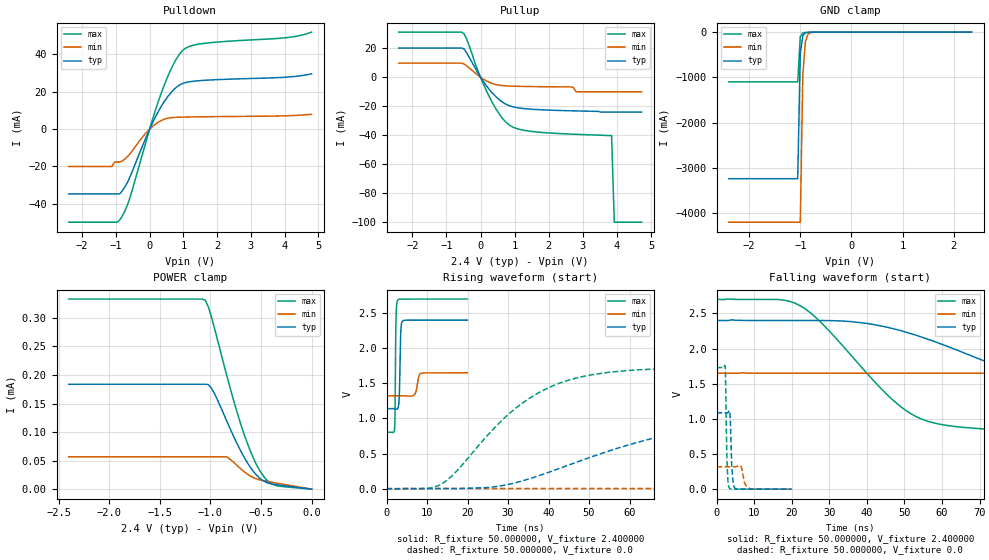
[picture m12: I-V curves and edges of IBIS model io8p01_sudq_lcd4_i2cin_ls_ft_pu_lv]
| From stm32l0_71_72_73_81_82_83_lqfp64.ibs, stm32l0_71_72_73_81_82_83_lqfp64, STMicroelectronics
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|   Model io8p01_sudq_lcd4_i2cin_ls_ft_pu_lv
[Model]  io8p01_sudq_lcd4_i2cin_ls_ft_pu_lv
Model_type I/O
Polarity   Non-Inverting
Enable   Active-Low
Vinl =   0.720000V
Vinh =   1.680000V
Vmeas =  1.200000V
Cref =   50.000000pF
Rref =   100.000000M
Vref =   0.0V
C_comp   2.470900pF   2.435200pF   2.490500pF
[Temperature Range]   25.000000   0.105000k   -40.000000
[Pullup Reference]   2.400000V   1.650000V   2.700000V
[Pulldown Reference]   0.0V   0.0V   0.0V
[POWER Clamp Reference]   2.400000V   1.650000V   2.700000V
[GND Clamp Reference]   0.0V   0.0V   0.0V
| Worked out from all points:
|   slope of the pulldown table from 0 to 0.36 V, typ, clamps not added: 28.5 ohm
|   slope of the pullup table from 0 to 0.36 V, typ, clamps not added: 32.2 ohm
|   GND clamp passes 1 mA (typ) near -0.64 V on its own axis
|   rising waveform, R_fixture 50.000000, V_fixture 2.400000: 20-80 % time 282ps typ, 636ps min, 192ps max; typ from 1.14 V to 2.4 V
|   rising waveform, R_fixture 50.000000, V_fixture 0.0: 20-80 % time 39.5ns typ, 107ns min, 19.3ns max; typ from 0.001 V to 1.09 V
|   falling waveform, R_fixture 50.000000, V_fixture 2.400000: 20-80 % time 40.8ns typ, 106ns min, 20.1ns max; typ from 2.4 V to 1.14 V
|   falling waveform, R_fixture 50.000000, V_fixture 0.0: 20-80 % time 457ps typ, 824ps min, 362ps max; typ from 1.09 V to 0.001 V
[Pulldown]
|Voltage   I(typ)   I(min)   I(max)
-2.4V     -34.71mA   -20mA      -49.82mA
-1.12V    -34.71mA   -20mA      -49.82mA
-1.04V    -34.71mA   -17.6mA    -49.82mA
-880mV    -34.55mA   -17.6mA    -48.46mA
-560mV    -24.65mA   -12.68mA   -35.33mA
0V        0A         0A         0A
400mV     13.84mA    5.066mA    22.03mA
720mV     21.25mA    6.254mA    35.26mA
1.04V     24.83mA    6.464mA    43.02mA
1.6V      26.11mA    6.627mA    45.88mA
4V        27.76mA    7.125mA    48.87mA
4.8V      29.64mA    7.94mA     51.96mA
[Pullup]
|Voltage   I(typ)   I(min)   I(max)
-2.4V     20.23mA    9.819mA    31.21mA
-480mV    19.53mA    9.213mA    29.94mA
0V        90fA       7.57pA     10fA
320mV     -10.16mA   -4.078mA   -16.34mA
640mV     -17.08mA   -5.718mA   -28.28mA
960mV     -20.45mA   -6.129mA   -34.49mA
1.76V     -22.39mA   -6.471mA   -37.97mA
2.64V     -23.11mA   -6.64mA    -39.19mA
2.8V      -23.2mA    -10mA      -39.35mA
3.84V     -24mA      -10mA      -40.2mA
3.92V     -24mA      -10mA      -100mA
4.72V     -24mA      -10mA      -100mA
[GND_clamp]
|Voltage   I(typ)   I(min)   I(max)
-2.4V     -3.237A    -4.197A    -1.1A
-1.05V    -3.237A    -4.197A    -1.1A
-1V       -475.5mA   -4.197A    -104.1mA
-950mV    -76.08mA   -935.1mA   -18.44mA
-900mV    -16.57mA   -212.6mA   -9.263mA
-850mV    -6.62mA    -50.88mA   -6.764mA
-800mV    -4.092mA   -13.84mA   -4.994mA
-650mV    -1.07mA    -1.21mA    -1.175mA
2.35V     0A         0A         0A
[POWER_clamp]
|Voltage   I(typ)   I(min)   I(max)
-2.4V     183.7uA    56.67uA    333uA
-1.05V    183.7uA    56.67uA    330.8uA
-1.02V    183.2uA    56.67uA    319.3uA
-960mV    167.4uA    56.67uA    282.2uA
-840mV    120.1uA    56.67uA    200.3uA
-750mV    84.75uA    43.78uA    142.9uA
-690mV    63.55uA    34.11uA    108.5uA
-600mV    37.04uA    22.45uA    64.63uA
-510mV    18.73uA    16.35uA    31.91uA
-450mV    12.06uA    14.02uA    17.25uA
-360mV    8.154uA    11.11uA    6.782uA
0V        0A         0A         0A
[Ramp]
| variable   typ   min   max
dV/dt_r  0.65095/39.48291n   0.19015/0.10644u   1.03799/19.28159n
dV/dt_f  0.75618/40.77217n   0.19446/0.10512u   1.13779/20.05274n
R_load = 50.000000
[Rising Waveform]
R_fixture= 50.000000
V_fixture= 2.400000
V_fixture_min= 1.650000
V_fixture_max= 2.700000
|time   V(typ)   V(min)   V(max)
0s        1.14V      1.323V     803.7mV
1.962ns   1.14V      1.323V     842.3mV
2.082ns   1.139V     1.323V     1.022V
2.362ns   1.135V     1.323V     2.455V
2.723ns   1.137V     1.323V     2.681V
3.163ns   1.343V     1.323V     2.698V
3.564ns   2.276V     1.323V     2.699V
3.924ns   2.384V     1.323V     2.699V
8.569ns   2.4V       1.642V     2.7V
19.94ns   2.4V       1.65V      2.7V
[Rising Waveform]
R_fixture= 50.000000
V_fixture= 0.0
V_fixture_min= 0.0
V_fixture_max= 0.0
|time   V(typ)   V(min)   V(max)
0s        880.8uV    1.332mV    514.1uV
14.01ns   2.455mV    2.472mV    83mV
29.03ns   49.24mV    2.472mV    1.002V
38.04ns   194.3mV    2.472mV    1.383V
48.05ns   400.8mV    2.474mV    1.592V
62.06ns   661.2mV    2.544mV    1.693V
95.1ns    980.6mV    5.941mV    1.728V
142.1ns   1.075V     80.7mV     1.73V
260.3ns   1.086V     274.1mV    1.73V
498.5ns   1.086V     318.6mV    1.73V
[Falling Waveform]
R_fixture= 50.000000
V_fixture= 2.400000
V_fixture_min= 1.650000
V_fixture_max= 2.700000
|time   V(typ)   V(min)   V(max)
0s        2.4V       1.65V      2.7V
21.02ns   2.4V       1.65V      2.643V
28.03ns   2.4V       1.65V      2.361V
50.05ns   2.24V      1.65V      1.133V
58.06ns   2.099V     1.65V      940.1mV
71.07ns   1.828V     1.65V      857.3mV
99.1ns    1.363V     1.65V      815.2mV
137.1ns   1.2V       1.635V     805.6mV
288.3ns   1.14V      1.381V     803.7mV
498.5ns   1.14V      1.323V     803.7mV
[Falling Waveform]
R_fixture= 50.000000
V_fixture= 0.0
V_fixture_min= 0.0
V_fixture_max= 0.0
|time   V(typ)   V(min)   V(max)
0s        1.086V     318.6mV    1.73V
2.282ns   1.086V     318.6mV    1.746V
2.402ns   1.086V     318.6mV    1.584V
2.843ns   1.085V     318.6mV    330.1mV
3.403ns   1.12V      318.6mV    18.74mV
3.644ns   1.014V     318.6mV    6.506mV
4.164ns   247.6mV    318.4mV    1.128mV
4.845ns   18.07mV    318.2mV    702.9uV
8.889ns   922.7uV    9.459mV    530.9uV
19.94ns   880.8uV    1.332mV    514.1uV
